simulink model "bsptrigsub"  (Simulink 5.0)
settings: Solver=ode45  SolverMode=SingleTasking  StartTime=0.0  StopTime=10.0  FixedStep=0.01  RelTol=1e-3

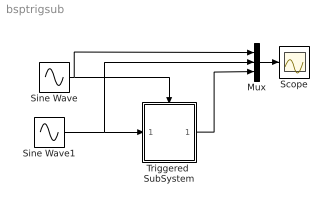
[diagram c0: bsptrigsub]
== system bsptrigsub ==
  Mux : Mux  Inputs=3
  Scope : Scope
  Sine Wave : Sin  Amplitude=0.2  Frequency=10  SampleTime=0
  Sine Wave1 : Sin  SampleTime=0
  Triggered  SubSystem : Subsystem
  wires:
  Sine Wave1/1 -> Triggered  SubSystem/1(In1), Mux/2
  Mux/1 -> Scope/1
  Sine Wave/1 -> Triggered  SubSystem/Trigger, Mux/1
  Triggered  SubSystem/1(Out1) -> Mux/3

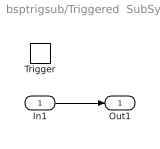
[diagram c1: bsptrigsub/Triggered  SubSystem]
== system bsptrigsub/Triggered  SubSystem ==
  In1 : Inport
  Trigger : TriggerPort  TriggerType=either
  Out1 : Outport
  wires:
  In1/1 -> Out1/1
